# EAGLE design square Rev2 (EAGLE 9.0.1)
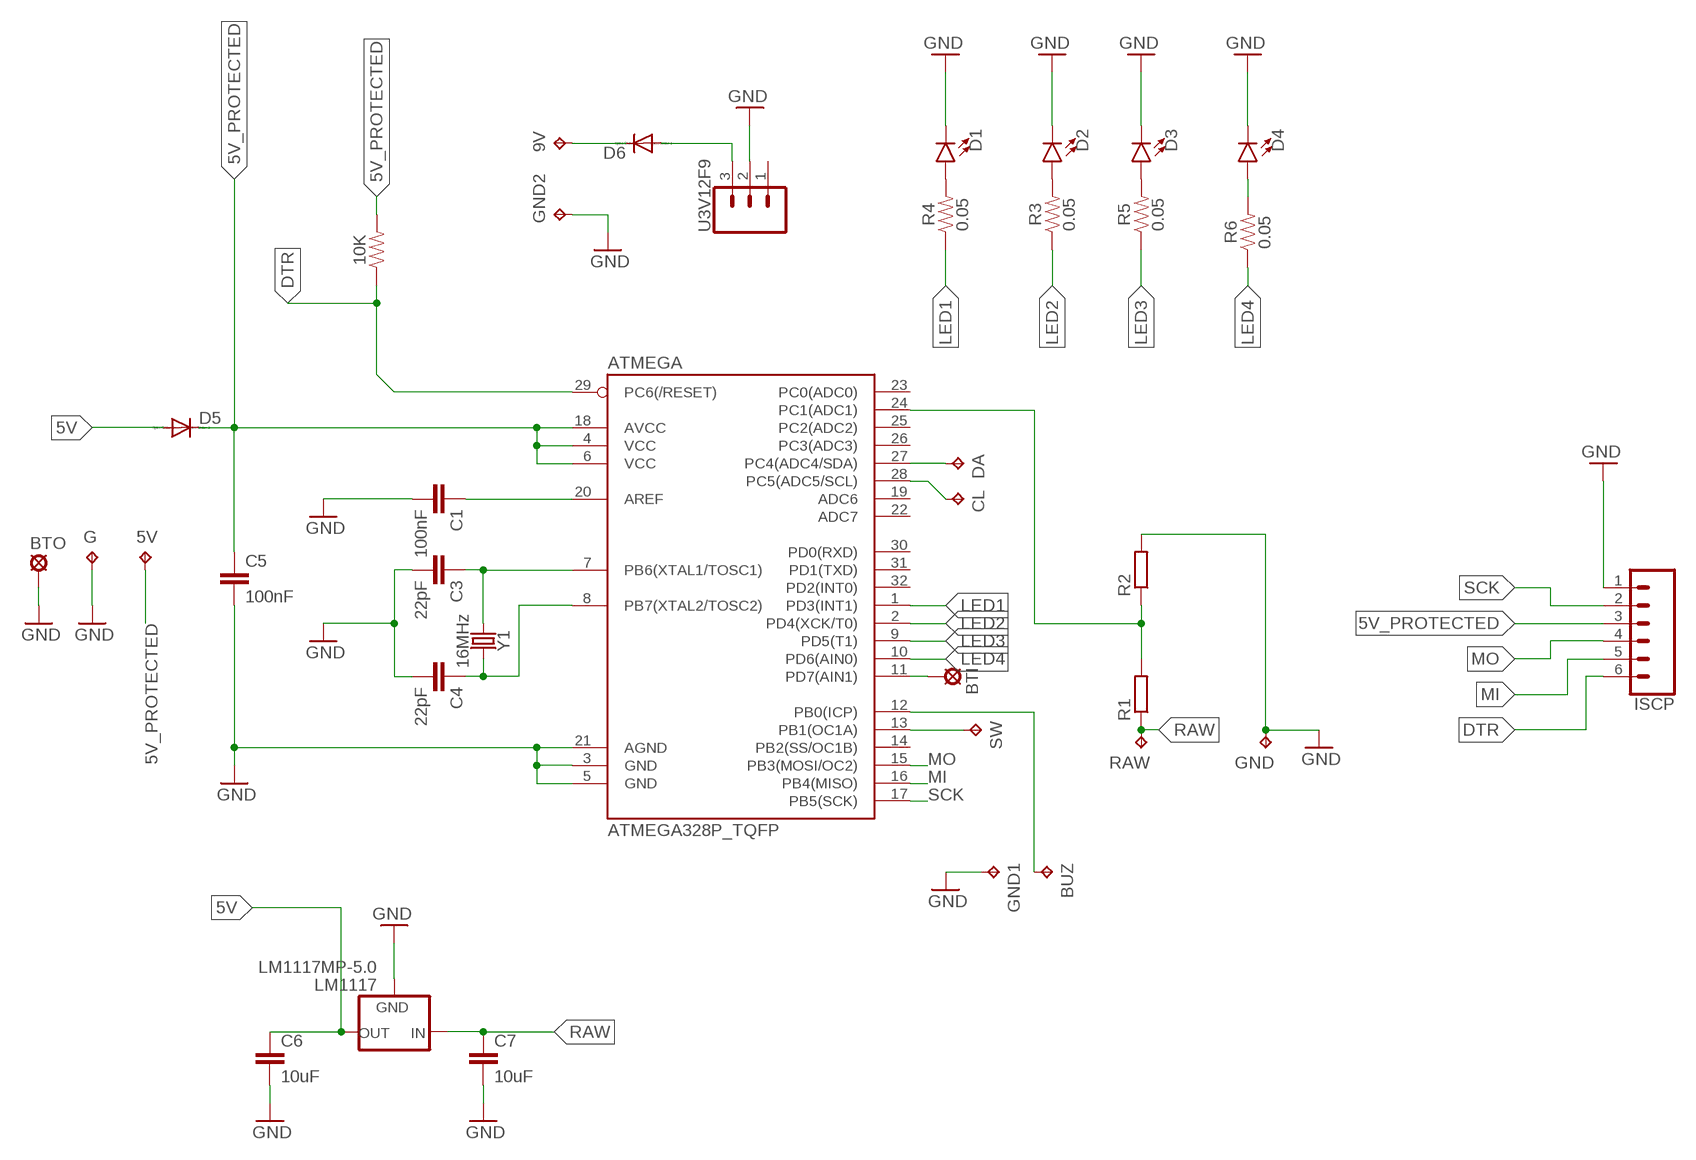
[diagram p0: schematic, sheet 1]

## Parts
5V  TPB1,27  [B1,27]
9V  TPB2,54  [B2,54]
10K  0.27OHM-0603-1/10W-1%  [0603]
ATMEGA  ATMEGA328P_TQFP  [TQFP32-08]
BTI  LSP10  [LSP10]
BTO  LSP10  [LSP10]
BUZ  TPB2,54  [B2,54]
C1  100nF  10NF-0603-50V-10%  [0603]
C3  22pF  10NF-0603-50V-10%  [0603]
C4  22pF  10NF-0603-50V-10%  [0603]
C5  100nF  10NF-0603-50V-10%  [0603]
C6  10uF  10NF-0603-50V-10%  [0603]
C7  10uF  10NF-0603-50V-10%  [0603]
CL  TPB1,27  [B1,27]
D1  LED1206  [LED-1206]
D2  LED1206  [LED-1206]
D3  LED1206  [LED-1206]
D4  LED1206  [LED-1206]
D5  DIODE-SOD106A-R  [SOD106A-R]
D6  DIODE-SOD106A-R  [SOD106A-R]
DA  TPB1,27  [B1,27]
G  TPB1,27  [B1,27]
GND  TPB2,54  [B2,54]
GND1  TPB2,54  [B2,54]
GND2  TPB2,54  [B2,54]
ISCP  CONN_06SMD-1MM  [1X06-1MM]
LM1117  LM1117MP-5.0  [SOT223]
R1  R-EU_R1206  [R1206]
R2  R-EU_R1206  [R1206]
R3  0.05  0.05OHM-0603-1/5W-1%  [0603]
R4  0.05  0.05OHM-0603-1/5W-1%  [0603]
R5  0.05  0.05OHM-0603-1/5W-1%  [0603]
R6  0.05  0.05OHM-0603-1/5W-1%  [0603]
RAW  TPB2,54  [B2,54]
SW  TPB1,27  [B1,27]
U3V12F9  CONN_03  [1X03]
Y1  16MHz  CRYSTALSMD-5X3.2-2PAD  [CRYSTAL-SMD-5X3.2-2PAD]

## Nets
5V [power]: C6.1 D5.A LM1117.2(OUT) LM1117.4(OUT)
5V_PROTECTED [power]: 5V.TP 10K.2 ATMEGA.4(VCC) ATMEGA.6(VCC) ATMEGA.18(AVCC) C5.1 D5.C ISCP.3
9VOUT [9v]: D6.A U3V12F9.3
AREF: ATMEGA.20(AREF) C1.1
BUZZER: ATMEGA.12(PB0(ICP)) BUZ.TP
DTR: 10K.1 ATMEGA.29(PC6(/RESET)) ISCP.6
GND [power]: ATMEGA.3(GND) ATMEGA.5(GND) ATMEGA.21(AGND) BTO.MP C1.2 C3.2 C4.2 C5.2 C6.2 C7.2 D1.C D2.C D3.C D4.C G.TP GND1.TP GND2.TP GND.TP ISCP.1 LM1117.1(GND) R2.2 U3V12F9.2
GREEN1: D2.A R3.2
GREEN2: D3.A R5.2
GREEN3: D4.A R6.2
LED1: ATMEGA.1(PD3(INT1)) R4.1
LED2: ATMEGA.2(PD4(XCK/T0)) R3.1
LED3: ATMEGA.9(PD5(T1)) R5.1
LED4: ATMEGA.10(PD6(AIN0)) R6.1
MI: ATMEGA.16(PB4(MISO)) ISCP.5
MO: ATMEGA.15(PB3(MOSI/OC2)) ISCP.4
N$2: ATMEGA.13(PB1(OC1A)) SW.TP
N$3: ATMEGA.11(PD7(AIN1)) BTI.MP
N$21 [9v]: 9V.TP D6.C
RAW [9v]: C7.1 LM1117.3(IN) R1.1 RAW.TP
RED: D1.A R4.2
SCK: ATMEGA.17(PB5(SCK)) ISCP.2
SCL: ATMEGA.28(PC5(ADC5/SCL)) CL.TP
SDA: ATMEGA.27(PC4(ADC4/SDA)) DA.TP
VOLTSENS: ATMEGA.24(PC1(ADC1)) R1.2 R2.1
XTAL1: ATMEGA.7(PB6(XTAL1/TOSC1)) C3.1 Y1.P$1
XTAL2: ATMEGA.8(PB7(XTAL2/TOSC2)) C4.1 Y1.P$2
Unconnected: ATMEGA.14(PB2(SS/OC1B)) ATMEGA.19(ADC6) ATMEGA.22(ADC7) ATMEGA.23(PC0(ADC0)) ATMEGA.25(PC2(ADC2)) ATMEGA.26(PC3(ADC3)) ATMEGA.30(PD0(RXD)) ATMEGA.31(PD1(TXD)) ATMEGA.32(PD2(INT0)) U3V12F9.1

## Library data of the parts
5V 9V BUZ CL DA G GND GND1 GND2 RAW SW = testpad:TP: Test pad
10K = SparkFun-Resistors:0.27OHM: 0.27Ω resistor; PROD_ID: RES-08787; VALUE: 0.27
ATMEGA = SparkFun-IC-Microcontroller:ATMEGA328P_TQFP: Popular 328P in QFP Storefront component: ATmega328 - TQFP (COM-13448) Datasheet SparkFun Products SparkFun RedBoard - Programmed with Arduino (DEV-12757) Arduino Pro Mini 328 - 5V/16MHz (DEV-11113) Arduino Pro Mini 328 - 3.3V/8MHz (DEV-11114) SparkFun OpenLog (DEV-13712) SparkFun MicroView - OLED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; PROD_ID: IC-09069
BTI BTO = solpad:LSP10: SOLDER PAD
C1 C3-C7 = SparkFun-Capacitors:10NF: 0.01uF/10nF/10,000pF ceramic capacitors; PROD_ID: CAP-00867; VALUE: 10nF
D1-D4 = SparkFun-LED:LED: LED (Generic)
D5 D6 = diode:DIODE-: DIODE
ISCP = SparkFun-Connectors:CONN_06: Multi connection point. Often used as Generic Header-pin footprint for 0.1 inch spaced/style header connections On any of the 0.1 inch spaced packages, you can populate with these: Break Away Headers - Straight (PRT-00116) Break Away Male Headers - Right Angle (PRT-00553) Female Headers (PRT-00115)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; PROD_ID: CONN-08249; SF_ID: GPS-00579
LM1117 = lm1117_10:LM1117?-*: 800mA Low-Dropout Linear Regulator Source: http://www.ti.com/lit/ds/symlink/lm1117-n.pdf; MF: Texas Instruments; MPN: LM1117MP-5.0; OC_FARNELL: 9778209; OC_NEWARK: 28X3417
R1 R2 = Clean-Kong:R-EU_: RESISTOR, European symbol
R3-R6 = SparkFun-Resistors:0.05OHM: 0.05Ω resistor; PROD_ID: RES-12535
U3V12F9 = SparkFun-Connectors:CONN_03: Multi connection point. Often used as Generic Header-pin footprint for 0.1 inch spaced/style header connections On any of the 0.1 inch spaced packages, you can populate with these: Break Away Headers - Straight (PRT-00116) Break Away Male Headers - Right Angle (PRT-00553) Female Headers (PRT-00115)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
Y1 = SparkFun-Clocks:CRYSTAL: Crystals (Generic)

## Module VCC
Ports: 

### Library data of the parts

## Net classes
0 default: width 0.2 mm, drill 0.254 mm, clearance 0.16 mm
1 power: width 0.3 mm, drill 0.3 mm, clearance 0.2 mm
2 9v: width 0.399 mm, drill 0.399 mm, clearance 0.3 mm

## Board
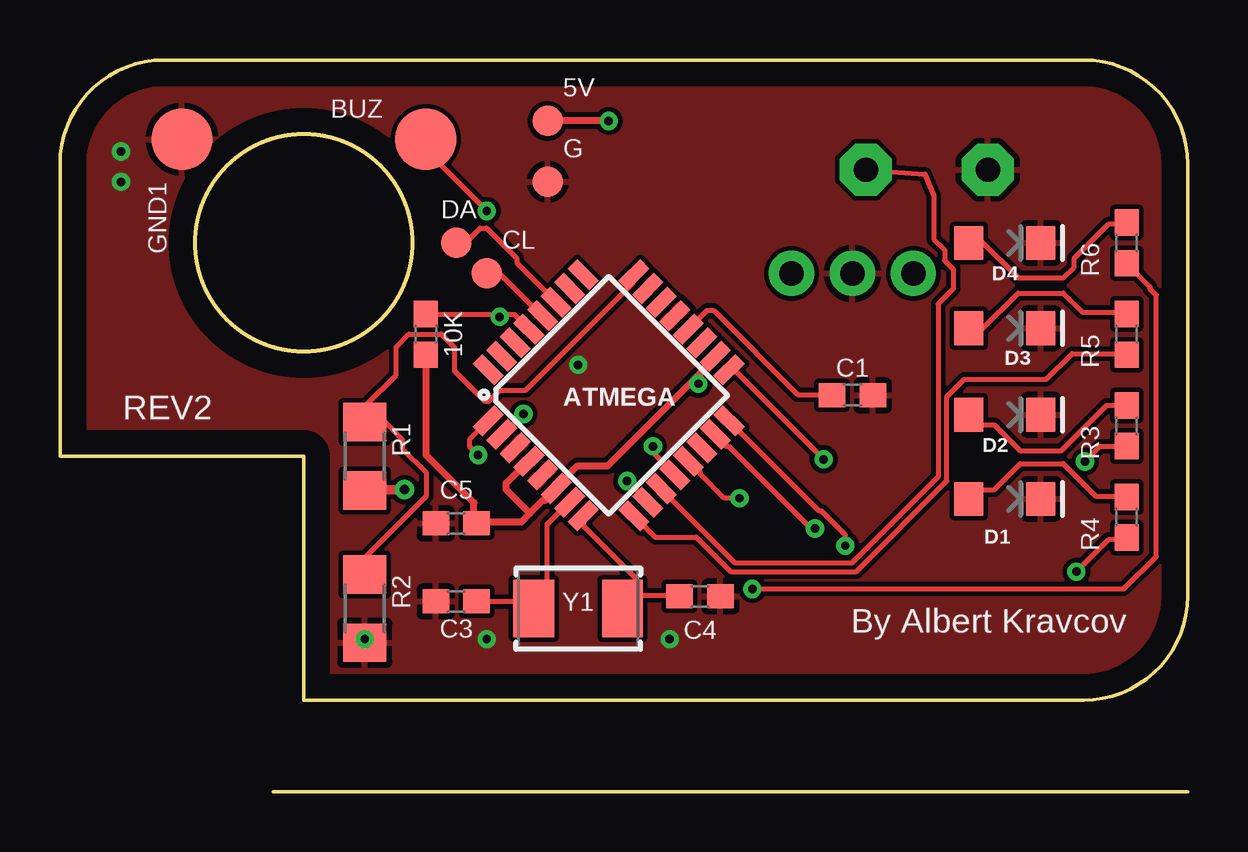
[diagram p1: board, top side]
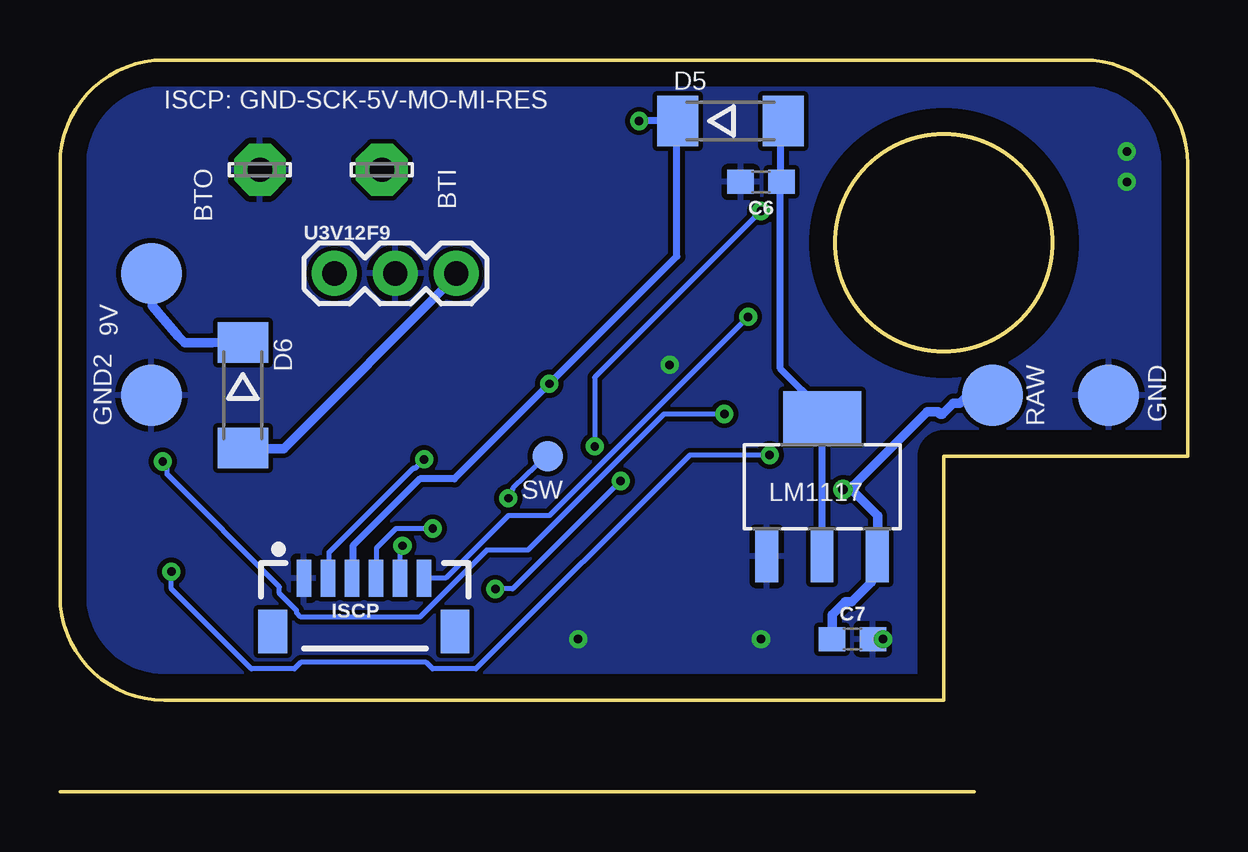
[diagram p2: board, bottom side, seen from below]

Size 46.99 x 30.48 mm. Coordinates in mm from the lower left corner, seen from the top.
Outline: 0,13.97 0,26.14 arc-90 4.34,30.48 42.65,30.48 arc-90 46.99,26.14 46.99,8.15 arc-90 42.65,3.81 10.16,3.81 10.16,13.97 0,13.97
Outline: circle at 10.16,22.86 radius 4.52
Copper layers (1*16): Top 0.035mm / dielectric 1.5mm / Bottom 0.035mm
Design rules "default *": minimum track width 6mil, minimum drill 0.35mm, track to track 6mil, track to pad 6mil, pad to pad 6mil, via to via 6mil, smd to smd 6mil, copper to edge 40mil, drill to drill 6mil, minimum pad ring 10mil, minimum via ring 8mil, stop-mask expansion 4mil, vias tented up to drill 2mm, thermal gap 10mil

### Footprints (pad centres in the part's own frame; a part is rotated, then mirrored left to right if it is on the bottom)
B1,27 = smd 1.27 x 1.27: TP 0,0
B2,54 = smd 2.54 x 2.54: TP 0,0
0603 = smd 1.1 x 1: 1 -0.85,0; 2 0.85,0
TQFP32-08 = smd 1.27 x 0.559: 1 -4.293,2.8; 2 -4.293,2; 3 -4.293,1.2; 4 -4.293,0.4; 5 -4.293,-0.4; 6 -4.293,-1.2; 7 -4.293,-2; 8 -4.293,-2.8; 17 4.293,-2.8; 18 4.293,-2; 19 4.293,-1.2; 20 4.293,-0.4; 21 4.293,0.4; 22 4.293,1.2; 23 4.293,2; 24 4.293,2.8 | smd 0.559 x 1.27: 9 -2.8,-4.293; 10 -2,-4.293; 11 -1.2,-4.293; 12 -0.4,-4.293; 13 0.4,-4.293; 14 1.2,-4.293; 15 2,-4.293; 16 2.8,-4.293; 25 2.8,4.293; 26 2,4.293; 27 1.2,4.293; 28 0.4,4.293; 29 -0.4,4.293; 30 -1.2,4.293; 31 -2,4.293; 32 -2.8,4.293
LSP10 = drill 1.016 pad 2.159 octagon: MP 0,0
LED-1206 = smd 1.2 x 1.4: A -1.5,0; C 1.5,0
SOD106A-R = smd 1.7 x 2.1: A 2.2,0; C -2.2,0
1X06-1MM = smd 0.6 x 1.55: 1 -2.54,1.27; 2 -1.54,1.27; 3 -0.54,1.27; 4 0.46,1.27; 5 1.46,1.27; 6 2.46,1.27 | smd 1.2 x 1.8: P$1 -3.84,-0.955; P$2 3.76,-0.955
SOT223 = smd 0.95 x 2.15: 1 -2.3,-2.9; 2 0,-2.9; 3 2.3,-2.9 | smd 3.25 x 2.15: 4 0,2.9
R1206 = smd 1.6 x 1.803: 1 -1.422,0; 2 1.422,0
1X03 = drill 1.016 pad 1.88: 1 0,0; 2 2.54,0; 3 5.08,0
CRYSTAL-SMD-5X3.2-2PAD = smd 1.7 x 2.4: P$1 1.85,0; P$2 -1.85,0

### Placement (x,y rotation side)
5V  20.32,27.94 0 top
9V  43.18,21.59 0 bottom
10K  15.24,19.05 270 top
ATMEGA  22.86,16.51 45 top
BTI  33.58,25.91 0 bottom
BTO  38.66,25.91 0 bottom
BUZ  15.24,27.18 90 top
C1  33.02,16.51 0 top
C3  16.51,7.92 180 top
C4  26.67,8.13 0 top
C5  16.51,11.18 180 top
C6  17.78,25.4 180 bottom
C7  13.97,6.35 0 bottom
CL  17.78,21.59 0 top
D1  39.37,12.19 0 top
D2  39.37,15.7 0 top
D3  39.37,19.3 0 top
D4  39.37,22.86 0 top
D5  19.05,27.94 0 bottom
D6  39.37,16.51 270 bottom
DA  16.51,22.86 0 top
G  20.32,25.4 0 top
GND  3.3,16.51 0 bottom
GND1  5.08,27.18 180 top
GND2  43.18,16.51 0 bottom
ISCP  34.29,7.62 0 bottom
LM1117  15.24,12.7 0 bottom
R1  12.7,13.97 90 top
R2  12.7,7.62 270 top
R3  44.45,15.24 90 top
R4  44.45,11.43 90 top
R5  44.45,19.05 90 top
R6  44.45,22.86 90 top
RAW  8.13,16.51 180 bottom
SW  26.67,13.97 180 bottom
U3V12F9  35.56,21.59 0 bottom
Y1  21.59,7.62 180 top

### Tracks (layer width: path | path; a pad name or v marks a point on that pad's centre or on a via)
5V
  Bottom 0.3: D5.A 16.88,27.88 16.97,27.79 16.97,25.45 C6.1 16.97,25.27 16.97,17.62 15.26,15.91 15.26,15.73 LM1117.4 15.26,15.55 15.26,9.88 LM1117.2
5V_PROTECTED  (via drill 0.35)
  Top 0.3: 19.58,11.59 20.12,12.13 20.21,12.13 20.66,12.58 ATMEGA.6 20.75,12.76 21.56,13.57 22.82,13.57 26.42,17.17 | 19.58,11.59 19.22,11.23 17.42,11.23 C5.1 17.24,11.23 17.24,12.04 15.26,14.02 15.26,18.16 10K.2 | 19.58,11.59 18.59,12.58 18.59,12.85 19.49,13.75 ATMEGA.4 | 26.42,17.17 26.87,17.62 26.87,17.71 27.23,18.07 ATMEGA.18 | v26.6,16.99 26.42,17.17 | v22.86,27.94 5V.TP
  Bottom 0.3: ISCP.3 34.79,8.89 34.79,10.24 32,13.03 30.56,13.03 v26.6,16.99 21.29,22.3 21.29,27.88 D5.C v22.86,27.94
9VOUT
  Bottom 0.399: D6.A 39.37,14.29 37.67,14.29 30.56,21.4 30.56,21.58 U3V12F9.3
AREF
  Top 0.2: C1.1 32.09,16.54 30.74,16.54 27.23,20.05 26.96,20.05 26.24,19.33 ATMEGA.20
BUZZER  (via drill 0.35)
  Top 0.2: v24.71,14.38 24.71,14.11 25.61,13.21 ATMEGA.12 | v17.78,24.19 15.26,26.71 15.26,27.16 BUZ.TP
  Bottom 0.2: v24.71,14.38 24.71,17.26 v17.78,24.19
DTR  (via drill 0.35)
  Top 0.2: 18.32,19.87 18.95,19.87 19.49,19.33 ATMEGA.29 | 18.32,19.87 15.26,19.87 10K.1 | v18.32,19.78 18.32,19.87
  Bottom 0.2: ISCP.6 30.92,8.89 28.31,11.5 26.6,11.5 v18.32,19.78
GND  (via drill 0.35)
  other vias: 12.7,6.35 17.78,6.35 21.59,17.78 2.54,26.67 2.54,25.4 25.4,6.35
  pour Top: -5.08,33.02 53.34,33.02 53.34,-2.54 -5.08,-2.54
  pour Bottom: -3.81,-2.54 -3.81,40.64 50.8,40.64 50.8,-2.54
GREEN1
  Top 0.2: R3.2 43.61,16.09 41.72,14.2 40.01,14.2 38.93,15.28 38.3,15.28 37.94,15.64 D2.A
GREEN2
  Top 0.2: R5.2 44.42,19.96 42.62,19.96 41.81,20.77 39.92,20.77 38.39,19.24 37.94,19.24 D3.A
GREEN3
  Top 0.2: R6.2 44.42,23.65 43.7,23.65 42.26,22.21 42.26,21.85 41.81,21.4 39.92,21.4 38.39,22.93 37.94,22.93 D4.A
LED1  (via drill 0.35)
  Top 0.2: v42.35,9.16 43.7,10.51 44.42,10.51 R4.1 | v17.42,14.02 17.06,14.38 17.06,14.65 17.78,15.37 ATMEGA.1
  Bottom 0.2: v42.35,9.16 42.35,8.44 39.02,5.11 37.22,5.11 36.95,5.38 31.73,5.38 31.46,5.11 29.66,5.11 20.75,14.02 v17.42,14.02
LED2  (via drill 0.35)
  Top 0.2: v42.71,13.75 43.34,14.38 44.42,14.38 R3.1 | v19.31,15.73 18.5,14.92 ATMEGA.2
  Bottom 0.2: v42.71,13.75 42.53,13.57 42.53,13.21 37.85,8.53 37.85,8.26 37.13,7.54 37.13,7.45 36.95,7.27 32,7.27 29.21,10.06 27.5,10.06 21.83,15.73 v19.31,15.73
LED3
  Top 0.2: R5.1 44.42,18.25 42.17,18.25 41.09,17.17 37.67,17.17 36.95,16.45 36.95,12.94 33.17,9.16 27.95,9.16 26.51,10.6 24.8,10.6 23.99,11.41 ATMEGA.9
LED4  (via drill 0.35)
  Top 0.2: v28.85,8.44 44.33,8.44 45.68,9.79 45.68,20.68 45.41,20.95 45.41,21.04 44.51,21.94 R6.1 | v23.63,12.94 24.44,12.13 ATMEGA.10
  Bottom 0.2: v28.85,8.44 28.13,8.44 v23.63,12.94
MI  (via drill 0.35)
  Top 0.2: v32.72,10.24 32.72,10.69 31.73,11.68 31.64,11.68 27.95,15.37 ATMEGA.16
  Bottom 0.2: v32.72,10.24 32.81,10.15 32.81,8.89 ISCP.5
MO  (via drill 0.35)
  Top 0.2: v31.46,10.96 31.28,10.96 27.86,14.38 27.77,14.38 27.32,14.83 ATMEGA.15
  Bottom 0.2: v31.46,10.96 32.99,10.96 33.8,10.15 33.8,8.89 ISCP.4
N$2  (via drill 0.35)
  Top 0.2: v28.31,12.22 27.68,12.22 26.69,13.21 26.69,13.3 26.24,13.75 ATMEGA.13
  Bottom 0.2: v28.31,12.22 28.12,12.63 26.67,14.04 SW.TP
N$3
  Top 0.2: ATMEGA.11 25.07,12.58 28.13,9.52 32.99,9.52 36.59,13.12 36.59,20.32 37.22,20.95 37.22,21.76 36.86,22.12 36.86,22.57 36.41,23.02 36.41,24.82 36.04,25.72 33.5,25.9 BTI.MP
N$21
  Bottom 0.399: D6.C 40.64,18.7 41.8,18.7 42.07,18.97 43.15,20.24 9V.TP
RAW  (via drill 0.4)
  Top 0.399: v14.36,12.58 12.74,12.58 R1.1
  Bottom 0.399: C7.1 14.81,6.37 14.81,7.36 14.27,7.9 14,7.9 13.19,8.71 13.19,9.61 13.01,9.79 LM1117.3 12.92,9.97 12.92,11.5 14,12.58 | 14,12.58 v14.36,12.58 | RAW.TP 8.15,16.45 9.23,16.45 9.5,16.18 9.77,16.18 10.22,15.73 10.31,15.73 10.4,15.82 10.85,15.82 13.91,12.76 14,12.58
RED
  Top 0.2: R4.2 44.42,12.31 43.16,12.31 41.81,13.66 40.01,13.66 38.93,12.58 38.3,12.58 37.94,12.22 D1.A
SCK  (via drill 0.35)
  Top 0.2: v31.82,13.84 28.13,17.53 27.95,17.53 ATMEGA.17
  Bottom 0.2: v31.82,13.84 32.18,13.48 32.27,13.48 35.78,9.97 35.78,8.89 ISCP.2
SCL
  Top 0.2: CL.TP 18.32,21.58 20.03,19.87 ATMEGA.28
SDA
  Top 0.2: ATMEGA.27 20.66,20.41 19.04,22.03 19.04,22.21 17.78,23.47 17.51,23.47 16.97,22.93 16.52,22.93 DA.TP
VOLTSENS
  Top 0.2: ATMEGA.24 23.9,21.49 23.9,21.22 19.4,16.72 18.32,16.72 17.87,16.27 17.69,16.27 16.43,17.53 16.43,18.52 15.89,19.06 14.54,19.06 14,18.52 14,17.35 12.74,16.09 12.74,15.46 R1.2 12.83,15.46 13.46,15.46 14.27,14.65 14.27,14.29 15.26,13.3 15.26,12.31 12.74,9.79 12.74,9.07 R2.1
XTAL1
  Top 0.2: C3.1 17.42,7.9 19.4,7.9 19.67,7.63 Y1.P$1 19.49,7.9 20.3,8.71 20.3,11.14 21.2,12.04 ATMEGA.7
XTAL2
  Top 0.2: C4.1 25.79,8.17 23.99,8.17 Y1.P$2 24.08,8.26 24.08,8.8 21.83,11.05 21.83,11.41 ATMEGA.8

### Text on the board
tPlace: REV2 | By Albert Kravcov
bPlace: ISCP: GND-SCK-5V-MO-MI-RES

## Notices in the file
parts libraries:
SparkFun-IC-Microcontroller: Licensing: Creative Commons ShareAlike 4.0 International - https://creativecommons.org/licenses/by-sa/4.0
